| TEXAS INSTRUMENTS INCORPORATED
| Standard Linear and Logic Group
| IBIS Model of SN74CB3Q3257
| 4-BIT 1-OF-2 MULTIPLEXER/DEMULTIPLEXER 2.5-v/3.3-v LOW-VOLTAGE FET BUS SWITCH
| This file contains package information for the following:
|  TVSOP 16-pin (DGV) package as [Component] CB3Q3257_DGV
|  SSOP 16-pin (DBQ) package as [Component] CB3Q3257_DBQ
|  TSSOP 16-pin (PW) package as [Component] CB3Q3257_PW
|  QFN 16-pin (RGY) package as [Component] CB3Q3257_RGY
| This device can be powered at the following Vccs:
|  3.3 volt Vcc
|  2.5 volt Vcc
| This file provides unique models under the [Model Selector] for each Vcc.
| For operation at a specific Vcc, select the appropriate model after each
| [Model Selector] keyword.
[IBIS Ver]   3.2
[Comment char]  |_char
[File Name]   sn74cb3q3257.ibs
[File Rev]   1.1 | x_die
[Date]   July 12, 2003
[Source]   Data created from TI-SPICE simulations at TI-SLL.
[Notes]   The following is an IBIS list for the CB3Q3257.
   Please contact sllibis@ti.com with questions and
   comments concerning SLL IBIS models.
   - Power-clamp data has been deleted since there is no
   power-clamp diode in the device.
[Disclaimer] Property of Texas Instruments Incorporated.  Unauthorized
   reproduction and/or distribution is strictly prohibited.
   This product is protected under copyright law.
   Created  2002, (C) Copyright  2002, Texas Instruments
   Incorporated, All Rights Reserved
   UNLESS THERE IS A SIGNED, WRITTEN AGREEMENT TO THE
   CONTRARY, TEXAS INSTRUMENTS (TI) IS PROVIDING THE IBIS
   MODELS  AND WITHOUT ANY WARRANTY, EXPRESSED OR
   IMPLIED.  TI assumes no liability for:
   1) the accuracy of the IBIS models provided to your
   company;
   2) the proper functioning of these IBIS Models in your
   design or for any resulting applications; or
   3) infringement of patents, copyrights or intellectual
   property rights resulting from your use of these IBIS
   models.
   TI provides IBIS Models as a service to our customers.
   You and your company shall not distribute, sell or give
   these models to anyone else without prior written
   permission from TI.
   TI reserves the right to make changes to our products or
   to discontinue any semiconductor product or service
   without notice, and advises our customers to obtain the
   latest version of relevant information to verify, before
   placing orders, that the information being relied on is
   current.
   Please be aware that your receipt and use of the IBIS
   information provided shall serve as acceptance of these
   terms and conditions.  If you do not accept these terms,
   you should return or destroy the IBIS models and any
   other accompanying information immediately.
| Component CB3Q3257_DBQ 16-pin SSOP
[Component]   CB3Q3257_DBQ
[Manufacturer]   Texas Instruments, Inc.
[Package]
|   typ   min   max
R_pkg   3.800e-02   2.700e-02   5.900e-02
L_pkg   2.353e-09   1.491e-09   4.500e-09
C_pkg   2.100e-13   6.400e-14   5.920e-13
[Pin]   signal_name   model_name   R_pin   L_pin   C_pin
1   S   CB3Q3257_IN   5.800e-02   4.450e-09   5.920e-13
2   1B1   CB3Q3257_IO   4.000e-02   1.930e-09   1.110e-13
3   1B2   CB3Q3257_IO   2.800e-02   1.538e-09   7.600e-14
4   1A   CB3Q3257_IOA   2.700e-02   1.491e-09   6.400e-14
5   2B1   CB3Q3257_IO   2.700e-02   1.491e-09   6.400e-14
6   2B2   CB3Q3257_IO   2.700e-02   1.506e-09   7.500e-14
7   2A   CB3Q3257_IOA   3.300e-02   1.922e-09   1.090e-13
8   GND   GND   5.900e-02   4.500e-09   5.880e-13
9   3A   CB3Q3257_IOA   5.800e-02   3.695e-09   4.140e-13
10   3B2   CB3Q3257_IO   3.400e-02   2.685e-09   2.820e-13
11   3B1   CB3Q3257_IO   2.900e-02   1.552e-09   7.700e-14
12   4A   CB3Q3257_IOA   2.800e-02   1.506e-09   6.500e-14
13   4B2   CB3Q3257_IO   2.700e-02   1.492e-09   6.400e-14
14   4B1   CB3Q3257_IO   2.800e-02   1.534e-09   7.600e-14
15   NOE   CB3Q3257_IN   4.000e-02   2.703e-09   2.840e-13
16   VCC   POWER   5.600e-02   3.645e-09   4.180e-13
| Component CB3Q3257_DGV 16-pin TVSOP
[Component]   CB3Q3257_DGV
[Manufacturer]   Texas Instruments, Inc.
[Package]
|   typ   min   max
R_pkg   3.900e-02   3.300e-02   4.500e-02
L_pkg   2.543e-09   2.320e-09   2.938e-09
C_pkg   3.860e-13   3.340e-13   4.490e-13
[Pin]   signal_name   model_name   R_pin   L_pin   C_pin
1   S   CB3Q3257_IN   3.500e-02   2.907e-09   4.170e-13
2   1B1   CB3Q3257_IO   4.200e-02   2.558e-09   4.460e-13
3   1B2   CB3Q3257_IO   3.800e-02   2.341e-09   3.450e-13
4   1A   CB3Q3257_IOA   3.800e-02   2.320e-09   3.340e-13
5   2B1   CB3Q3257_IO   3.900e-02   2.322e-09   3.340e-13
6   2B2   CB3Q3257_IO   3.800e-02   2.353e-09   3.420e-13
7   2A   CB3Q3257_IOA   4.000e-02   2.536e-09   4.410e-13
8   GND   GND   3.300e-02   2.897e-09   4.180e-13
9   3A   CB3Q3257_IOA   3.500e-02   2.927e-09   4.190e-13
10   3B2   CB3Q3257_IO   4.500e-02   2.632e-09   4.490e-13
11   3B1   CB3Q3257_IO   3.900e-02   2.368e-09   3.470e-13
12   4A   CB3Q3257_IOA   3.900e-02   2.330e-09   3.350e-13
13   4B2   CB3Q3257_IO   3.900e-02   2.320e-09   3.350e-13
14   4B1   CB3Q3257_IO   3.900e-02   2.361e-09   3.450e-13
15   NOE   CB3Q3257_IN   4.100e-02   2.573e-09   4.460e-13
16   VCC   POWER   3.500e-02   2.938e-09   4.200e-13
| Component CB3Q3257_PW 16-pin TSSOP
[Component]   CB3Q3257_PW
[Manufacturer]   Texas Instruments, Inc.
[Package]
|   typ   min   max
R_pkg   4.500e-02   3.800e-02   5.100e-02
L_pkg   2.593e-09   2.447e-09   3.080e-09
C_pkg   2.810e-13   2.430e-13   3.770e-13
[Pin]   signal_name   model_name   R_pin   L_pin   C_pin
1   S   CB3Q3257_IN   4.000e-02   3.080e-09   3.770e-13
2   1B1   CB3Q3257_IO   3.800e-02   2.458e-09   2.810e-13
3   1B2   CB3Q3257_IO   5.100e-02   2.512e-09   2.550e-13
4   1A   CB3Q3257_IOA   5.100e-02   2.447e-09   2.430e-13
5   2B1   CB3Q3257_IO   5.100e-02   2.447e-09   2.430e-13
6   2B2   CB3Q3257_IO   5.100e-02   2.512e-09   2.550e-13
7   2A   CB3Q3257_IOA   3.800e-02   2.458e-09   2.810e-13
8   GND   GND   4.000e-02   3.080e-09   3.770e-13
9   3A   CB3Q3257_IOA   3.900e-02   2.832e-09   3.160e-13
10   3B2   CB3Q3257_IO   3.800e-02   2.460e-09   2.790e-13
11   3B1   CB3Q3257_IO   5.100e-02   2.512e-09   2.550e-13
12   4A   CB3Q3257_IOA   5.100e-02   2.447e-09   2.430e-13
13   4B2   CB3Q3257_IO   5.100e-02   2.447e-09   2.430e-13
14   4B1   CB3Q3257_IO   5.100e-02   2.512e-09   2.550e-13
15   NOE   CB3Q3257_IN   3.800e-02   2.459e-09   2.790e-13
16   VCC   POWER   3.900e-02   2.832e-09   3.160e-13
| Component CB3Q3257_RGY 16-pin QFN
[Component]   CB3Q3257_RGY
[Manufacturer]   Texas Instruments, Inc.
[Package]
|   typ   min   max
R_pkg   3.000e-02   2.700e-02   3.800e-02
L_pkg   8.000e-10   7.220e-10   9.400e-10
C_pkg   1.410e-13   1.290e-13   1.550e-13
[Pin]   signal_name   model_name   R_pin   L_pin   C_pin
1   S   CB3Q3257_IN   2.700e-02   8.180e-10   1.320e-13
2   1B1   CB3Q3257_IO   2.700e-02   8.030e-10   1.300e-13
3   1B2   CB3Q3257_IO   3.700e-02   9.080e-10   1.500e-13
4   1A   CB3Q3257_IOA   2.900e-02   7.220e-10   1.390e-13
5   2B1   CB3Q3257_IO   2.900e-02   7.220e-10   1.390e-13
6   2B2   CB3Q3257_IO   2.900e-02   7.300e-10   1.400e-13
7   2A   CB3Q3257_IOA   2.900e-02   7.240e-10   1.390e-13
8   GND   GND   3.100e-02   8.000e-10   1.400e-13
9   3A   CB3Q3257_IOA   2.700e-02   8.110e-10   1.290e-13
10   3B2   CB3Q3257_IO   2.800e-02   7.840e-10   1.310e-13
11   3B1   CB3Q3257_IO   3.700e-02   9.150e-10   1.530e-13
12   4A   CB3Q3257_IOA   2.900e-02   8.470e-10   1.520e-13
13   4B2   CB3Q3257_IO   2.900e-02   7.580e-10   1.430e-13
14   4B1   CB3Q3257_IO   2.900e-02   7.720e-10   1.440e-13
15   NOE   CB3Q3257_IN   2.900e-02   7.400e-10   1.420e-13
16   VCC   POWER   3.800e-02   9.400e-10   1.550e-13
[Series Switch Groups]
| Function Group States
On  1 /   | 1A->1B1 NOE LOW S LOW
   | 2A->2B1 NOE LOW S LOW
   | 3A->3B1 NOE LOW S LOW
   | 4A->4B1 NOE LOW S LOW
On  2 /   | 1A->1B2 NOE LOW S HIGH
   | 2A->2B2 NOE LOW S HIGH
   | 3A->3B2 NOE LOW S HIGH
   | 4A->4B2 NOE LOW S HIGH
Off 1 2 /   | NOE HIGH
[Series Pin Mapping]   pin_2   model_name   function_table_group
4   2   CB3Q3257_IOA_33_S   1
| 4   2   CB3Q3257_IOA_25_S   1
7   5   CB3Q3257_IOA_33_S   1
| 7   5   CB3Q3257_IOA_25_S   1
9   11   CB3Q3257_IOA_33_S   1
| 9   11   CB3Q3257_IOA_25_S   1
12   14   CB3Q3257_IOA_33_S   1
| 12   14   CB3Q3257_IOA_25_S   1
4   3   CB3Q3257_IOA_33_S   2
| 4   3   CB3Q3257_IOA_25_S   2
7   6   CB3Q3257_IOA_33_S   2
| 7   6   CB3Q3257_IOA_25_S   2
9   10   CB3Q3257_IOA_33_S   2
| 9   10   CB3Q3257_IOA_25_S   2
12   13   CB3Q3257_IOA_33_S   2
| 12   13   CB3Q3257_IOA_25_S   2
| Model CB3Q3257_IN
[Model Selector]   CB3Q3257_IN
CB3Q3257_IN_33   3.3 volt Vcc
CB3Q3257_IN_25   2.5 volt Vcc
| Model CB3Q3257_IOA
[Model Selector]   CB3Q3257_IOA
CB3Q3257_IOA_33   3.3 volt Vcc
CB3Q3257_IOA_25   2.5 volt Vcc
| Model CB3Q3257_IOA_S
[Model Selector]   CB3Q3257_IOA_S
CB3Q3257_IOA_33_S   3.3 volt Vcc
CB3Q3257_IOA_25_S   2.5 volt Vcc
| Model CB3Q3257_IO
[Model Selector]   CB3Q3257_IO
CB3Q3257_IO_33   3.3 volt Vcc
CB3Q3257_IO_25   2.5 volt Vcc
| Model CB3Q3257_IO_S
[Model Selector]   CB3Q3257_IO_S
CB3Q3257_IO_33_S   3.3 volt Vcc
CB3Q3257_IO_25_S   2.5 volt Vcc
[Model]   CB3Q3257_IOA_33_S
Model_type  Series_switch
| variable   typ   min   max
C_comp   0   0   0
[Temperature Range]   40   100   -40
| Ambient temperature   25   85   -40
[Voltage range]   3.3   3   3.6
[On]
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[Off]
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[Model]   CB3Q3257_IOA_25_S
Model_type  Series_switch
| variable   typ   min   max
C_comp   0   0   0
[Temperature Range]   40   100   -40
| Ambient temperature   25   85   -40
[Voltage range]   2.5   2.3   2.7
[On]
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[Off]
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[Model]   CB3Q3257_IO_33_S
Model_type  Series_switch
| variable   typ   min   max
C_comp   0   0   0
[Temperature Range]   40   100   -40
| Ambient temperature   25   85   -40
[Voltage range]   3.3   3   3.6
[On]
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[Off]
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[Model]   CB3Q3257_IO_25_S
Model_type  Series_switch
| variable   typ   min   max
C_comp   0   0   0
[Temperature Range]   40   100   -40
| Ambient temperature   25   85   -40
[Voltage range]   2.5   2.3   2.7
[On]
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[Off]
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| Models and submodels in the file (10): CB3Q3257_IN_33 (Input), CB3Q3257_IN_25 (Input), CB3Q3257_IOA_33_S (Series_switch), CB3Q3257_IOA_33 (Terminator), CB3Q3257_IOA_25_S (Series_switch), CB3Q3257_IOA_25 (Terminator), CB3Q3257_IO_33_S (Series_switch), CB3Q3257_IO_33 (Terminator), CB3Q3257_IO_25_S (Series_switch), CB3Q3257_IO_25 (Terminator)
